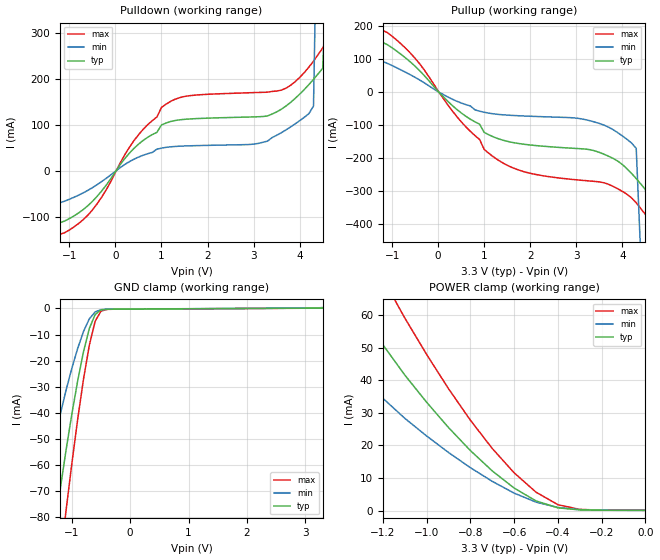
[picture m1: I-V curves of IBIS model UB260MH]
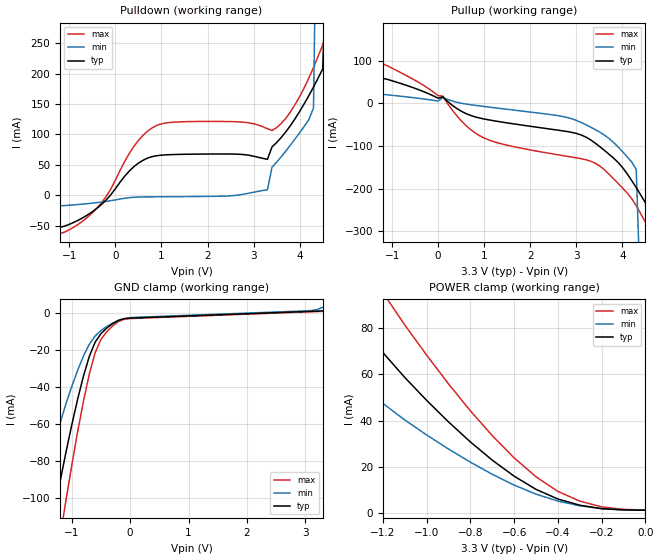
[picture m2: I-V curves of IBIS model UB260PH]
| IBIS file ub260omh.ibs created by s2ibis2 version 1.1
| North Carolina State University Electronics Research Laboratory  1995
[IBIS ver]   2.1
[File name]   z6usb11h.ibs
[File Rev]   1.0
[Date]   Monday, April 22, 2002
[Source]   From silicon level SPICE at TOSHIBA.
[Notes]   This model does not include the values of Package Model
[Disclaimer]   None.
[Copyright]   Copyright(C) TOSHIBA Corp. 1996-1998. All Rights Reserved
|   Component TC260C
[Component]   TC260C
[Manufacturer]   TOSHIBA
[Package]
| variable   typ   min   max
R_pkg   1.0000f   NA   NA
L_pkg   1.0000fH   NA   NA
C_pkg   1.0000fF   NA   NA
[Pin]  signal_name   model_name   R_pin   L_pin   C_pin
DM   DM   UB260MH
DP   DP   UB260PH
VDDS   VDDS   POWER
VSS   VSS   GND
| Models and submodels in the file (2): UB260MH (3-state), UB260PH (3-state)
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|   Model UB260MH
[Model]   UB260MH
Model_type   3-state
Polarity   Non-Inverting
C_comp   7.964pF   NA   NA
|Variable   typ   min   max
[Voltage range]  3.3   3.0   3.6
[Temperature Range]   25.0000   100.0000   0.000
[Pullup Reference]   3.3000V   3.0000V   3.6000V
[Pulldown Reference]   0.000V   0.000V   0.000V
[POWER Clamp Reference]   3.3000V   3.0000V   3.6000V
[GND Clamp Reference]   0.000V   0.000V   0.000V
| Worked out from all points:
|   slope of the pulldown table from 0 to 0.495 V, typ, clamps not added: 8.35 ohm
|   slope of the pullup table from 0 to 0.495 V, typ, clamps not added: 7.68 ohm
|   GND clamp passes 1 mA (typ) near -0.52 V on its own axis
|   POWER clamp passes 1 mA (typ) near -0.41 V on its own axis
[Pulldown]
| voltage   I(typ)   I(min)   I(max)
-3.3V     -5.02mA    -3.01mA    -9.23mA
-1.7V     -14.59mA   -12.91mA   -16.78mA
-1.5V     -36.55mA   -36.35mA   -39.3mA
-1.3V     -116.5mA   -72.87mA   -141.9mA
-500mV    -66.74mA   -36.87mA   -85.54mA
1.2V      107.3mA    52.14mA    151.2mA
3.3V      119.3mA    64.47mA    171.1mA
4.1V      177mA      116.4mA    213.9mA
4.3V      198.9mA    141mA      238.7mA
4.5V      223.2mA    1.27A      267.5mA
4.7V      691.1mA    5.084A     299.9mA
6.6V      45.54A     50.9A      38.97A
[Pullup]
| voltage   I(typ)   I(min)   I(max)
-3.3V     25.93mA    10.06mA    58.58mA
-1.7V     21.39mA    24.32mA    29.65mA
-1.5V     46.57mA    47.87mA    52.83mA
-1.3V     157.5mA    99.23mA    194mA
-600mV    91.68mA    52.99mA    118.5mA
1.4V      -144.8mA   -68.05mA   -213.6mA
3.2V      -172mA     -82.93mA   -267.6mA
4.2V      -246mA     -153.7mA   -320.1mA
4.3V      -261.4mA   -170mA     -334.6mA
4.5V      -294.4mA   -831.6mA   -370.2mA
4.7V      -566.9mA   -3.073A    -409.9mA
6.6V      -26.81A    -29.99A    -22.93A
[GND_clamp]
| voltage   I(typ)   I(min)   I(max)
-3.3V     -26.62A    -25.55A    -26.99A
-1.4V     -356.8mA   -160.3mA   -479.8mA
-1.3V     -95.09mA   -55.74mA   -129.5mA
-1.2V     -69.39mA   -40.75mA   -96.7mA
-1.1V     -54.4mA    -31.41mA   -77.57mA
-900mV    -27.78mA   -15.34mA   -42.49mA
-800mV    -16.59mA   -8.835mA   -27.11mA
-700mV    -7.701mA   -3.996mA   -14.1mA
-600mV    -2.328mA   -1.35mA    -4.928mA
-500mV    -587.6uA   -485.2uA   -1.043mA
-400mV    -332.4uA   -312.2uA   -385.5uA
3.3V      125.4uA    325.2uA    101.4uA
[POWER_clamp]
| voltage   I(typ)   I(min)   I(max)
-3.3V     45.19A     43.36A     45.82A
-1.4V     532.1mA    217.5mA    733.1mA
-1.3V     78.89mA    49.47mA    109.4mA
-1.2V     50.88mA    34.47mA    71.25mA
-1.1V     41.61mA    28.34mA    59.1mA
-900mV    25.5mA     17.85mA    37.41mA
-800mV    18.45mA    13.19mA    27.75mA
-600mV    6.945mA    5.392mA    11.62mA
-500mV    2.994mA    2.631mA    5.681mA
-400mV    883.9uA    999.3uA    1.844mA
-300mV    246.7uA    325.2uA    406uA
0V        125.4uA    114uA      136.8uA
[Ramp]
| variable   typ   min   max
dV/dt_r   1.7443/9.8841n   1.4353/10.7693n   1.9700/9.8054n
dV/dt_f   1.7040/10.4314n   1.3314/11.8715n   1.9426/10.2087n
R_load = 50.0000
| End [Model] UB260MH
|   Model UB260PH
[Model]   UB260PH
Model_type   3-state
Polarity   Non-Inverting
C_comp   7.914pF   NA   NA
|Variable   typ   min   max
[Voltage range]  3.3   3.0   3.6
[Temperature Range]   25.0000   100.0000   0.000
[Pullup Reference]   3.3000V   3.0000V   3.6000V
[Pulldown Reference]   0.000V   0.000V   0.000V
[POWER Clamp Reference]   3.3000V   3.0000V   3.6000V
[GND Clamp Reference]   0.000V   0.000V   0.000V
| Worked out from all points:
|   slope of the pulldown table from 0 to 0.495 V, typ, clamps not added: 11.9 ohm
|   slope of the pullup table from 0 to 0.495 V, typ, clamps not added: 16.5 ohm
[Pulldown]
| voltage   I(typ)   I(min)   I(max)
-3.3V     12.27mA    -8.69mA    30.59mA
-1.7V     4.589mA    -9.327mA   17.5mA
-1.5V     -8.083mA   -12.38mA   2.538mA
-1.3V     -54.22mA   -17.49mA   -64.98mA
-400mV    -21.09mA   -11.86mA   -20.75mA
900mV     65.21mA    -2.347mA   115mA
3.3V      59.21mA    9.249mA    109.5mA
3.4V      79.63mA    46.35mA    106.5mA
4.3V      177.9mA    143.6mA    209.9mA
4.5V      207.5mA    1.249A     247mA
4.7V      668.2mA    5.053A     287.8mA
6.6V      45.47A     50.82A     38.92A
[Pullup]
| voltage   I(typ)   I(min)   I(max)
-3.3V     75.58mA    19.78mA    177.4mA
-2.1V     29.21mA    9.24mA     66.81mA
-1.5V     30.36mA    13.99mA    52.69mA
-1.3V     61.68mA    22.36mA    97.29mA
100mV     15.55mA    14.09mA    17.27mA
1V        -36.5mA    -7.087mA   -81.18mA
2.9V      -67.81mA   -35.95mA   -125.8mA
4.2V      -180.6mA   -137.2mA   -223.2mA
4.3V      -197.4mA   -154.7mA   -239.8mA
4.5V      -233mA     -809.2mA   -278.8mA
4.7V      -499.5mA   -3.047A    -321.1mA
6.6V      -26.74A    -29.97A    -22.83A
[GND_clamp]
| voltage   I(typ)   I(min)   I(max)
-3.3V     -26.62A    -25.55A    -26.99A
-1.4V     -372mA     -177.4mA   -494.7mA
-1.3V     -117mA     -74.95mA   -153.8mA
-1.2V     -91.08mA   -59.3mA    -121.1mA
-1.1V     -75.28mA   -49.05mA   -101.3mA
-800mV    -33.98mA   -23.17mA   -47.58mA
-700mV    -23.36mA   -16.83mA   -32.86mA
-600mV    -15.65mA   -12.29mA   -21.33mA
-500mV    -11.04mA   -9.313mA   -14.17mA
-200mV    -3.821mA   -3.933mA   -4.463mA
3.1V      1.04mA     1.479mA    802.5uA
3.3V      1.279mA    3.2mA      1.041mA
[POWER_clamp]
| voltage   I(typ)   I(min)   I(max)
-3.3V     45.19A     43.37A     45.82A
-1.4V     545mA      230.1mA    746.8mA
-1.3V     98.26mA    63.28mA    134mA
-1.2V     69.33mA    47.4mA     95.18mA
-1.1V     58.58mA    40.24mA    81.25mA
-800mV    30.75mA    22.01mA    44.18mA
-600mV    15.98mA    12.14mA    23.88mA
-500mV    10.28mA    8.226mA    15.71mA
-400mV    6.119mA    5.237mA    9.405mA
-300mV    3.442mA    3.2mA      5.23mA
-200mV    1.946mA    1.996mA    2.727mA
0V        1.279mA    1.289mA    1.405mA
[Ramp]
| variable   typ   min   max
dV/dt_r   1.7443/9.8503n   1.4353/10.7506n   1.9699/9.7206n
dV/dt_f   1.7040/10.3095n   1.3316/11.7043n   1.9426/10.1004n
R_load = 50.0000
| End [Model] UB260PH
| End [Component] TC260C
